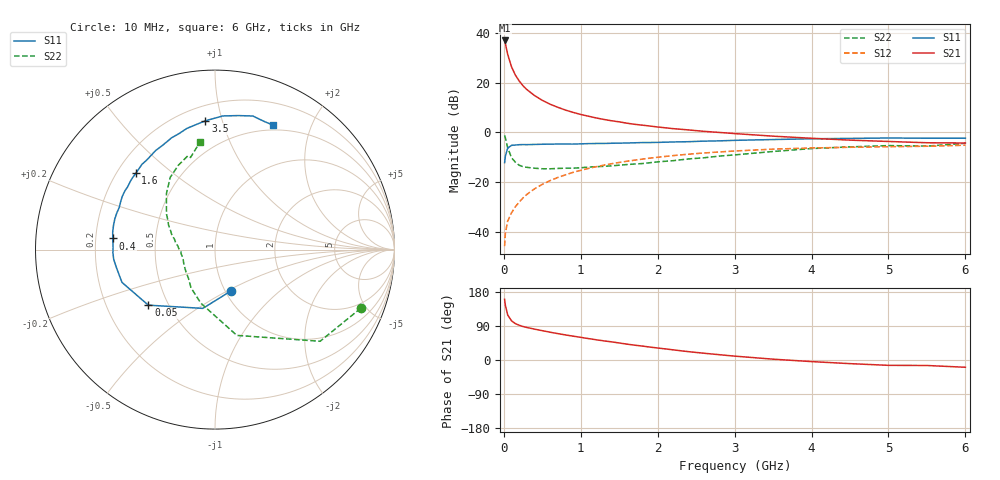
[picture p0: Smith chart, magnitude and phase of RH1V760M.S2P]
! SIEMENS Small Signal Semiconductors
! BFR106
! Si NPN RF Bipolar Junction Transistor in SOT23
! VCE = 1.75 V  IC = 60 mA
! Common Emitter S-Parameters:  August  1996
# GHz  S  MA  R  50
!  f  S11  S21  S12  S22
! GHz  MAG  ANG  MAG  ANG  MAG  ANG  MAG  ANG
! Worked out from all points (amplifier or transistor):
!   36 points, 10 MHz to 6 GHz, reference 50 ohm
!   highest |S21| = 37.1 dB at 10 MHz (marker M1)
!   |S21| within 3 dB of that: start of sweep to 31.84 MHz
!   unconditionally stable (mu >= 1): 200.3 MHz to 2.892 GHz; 5.023 GHz to end of sweep
!   at 250 MHz: K = 1.04, MAG = 21.4 dB, |S12| = -26.4 dB
!   at 1.4 GHz: K = 1.07, MAG = 7.1 dB, |S12| = -12.6 dB
!   at 6 GHz: K = 1.01, MAG = -0.3 dB, |S12| = -5.1 dB
!   S11 on the Smith chart (normalised r, x): 10 MHz: 1.07, -0.52; 50 MHz: 0.39, -0.31; 400 MHz: 0.27, +0.05; 1.6 GHz: 0.28, +0.38; 3.5 GHz: 0.30, +0.88; 6 GHz: 0.44, +1.48
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0.01  0.2464 -68.1  71.55 159.9  0.0051 77.4  0.8754 -21.9
0.02  0.3345 -101.7  61.62 144.4  0.0094 64.3  0.777 -41.1
0.05  0.4835 -140.2  37.51 118.8  0.0163 58.4  0.4933 -75.7
0.1  0.5496 -160.6  21.02 103.3  0.024 62.5  0.3091 -104.7
0.15  0.5582 -169.6  14.32 96.0  0.0319 65.6  0.2515 -122.1
0.2  0.5669 -174.5  10.9 91.7  0.0396 67.8  0.2181 -132.6
0.25  0.5693 -178.2  8.713 88.3  0.048 69.6  0.2042 -142.0
0.3  0.5678 179.1  7.297 85.8  0.0565 71.1  0.198 -147.5
0.4  0.573 173.8  5.53 81.4  0.0733 71.4  0.19 -156.7
0.5  0.5783 170.2  4.438 77.4  0.09 71.1  0.1855 -162.9
0.6  0.5815 166.4  3.717 73.4  0.1068 70.3  0.1851 -166.6
0.7  0.5838 162.9  3.221 69.7  0.1234 69.1  0.1881 -170.3
0.9  0.5828 156.4  2.539 62.9  0.1569 66.4  0.1905 -176.8
1.1  0.5957 150.2  2.124 56.5  0.1882 63.3  0.2003 179.3
1.3  0.5993 144.3  1.83 50.5  0.2193 59.9  0.2073 174.5
1.6  0.6124 136.1  1.537 41.9  0.2629 54.8  0.2253 168.9
2.2  0.6432 121.0  1.194 26.8  0.3413 44.3  0.2698 156.7
2.8  0.6764 107.3  1.001 14.0  0.4043 34.1  0.3337 144.0
3.5  0.7197 94.3  0.842 2.2  0.4606 23.1  0.4131 130.9
4.5  0.7582 80.0  0.7 -9.6  0.5023 9.0  0.5122 113.5
5.5  0.7647 68.8  0.62 -14.5  0.5269 0.5  0.531 104.9
6  0.7651 65.0  0.613 -19.2  0.553 -6.2  0.6029 98.1
